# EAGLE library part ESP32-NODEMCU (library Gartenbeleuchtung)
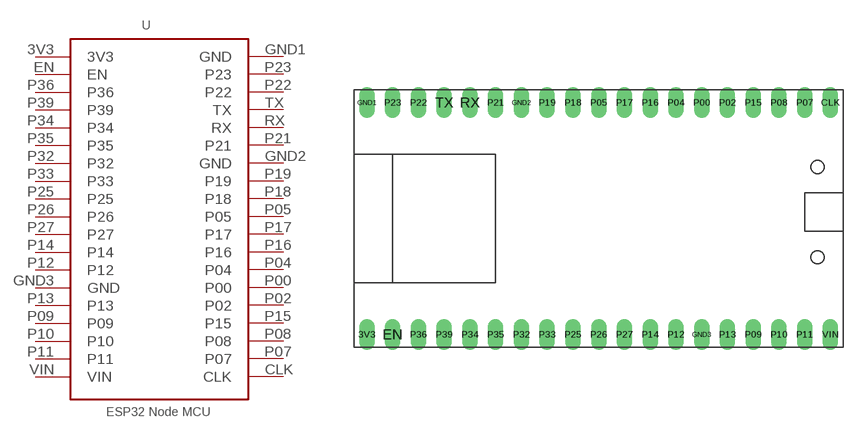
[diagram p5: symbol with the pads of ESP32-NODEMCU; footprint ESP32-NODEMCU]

Designator prefix -

## ESP32-NODEMCU  [ESP32-NODEMCU]
3V3  3V3  pwr
CLK  CLK
EN  EN
GND1  GND  pwr
GND2  GND  pwr
GND3  GND  pwr
P00  P00
P02  P02
P04  P04
P05  P05
P07  P07
P08  P08
P09  P09
P10  P10
P11  P11
P12  P12
P13  P13
P14  P14
P15  P15
P16  P16
P17  P17
P18  P18
P19  P19
P21  P21
P22  P22
P23  P23
P25  P25
P26  P26
P27  P27
P32  P32
P33  P33
P34  P34
P35  P35
P36  P36
P39  P39
RX  RX
TX  TX
VIN  VIN  pwr

## Footprint ESP32-NODEMCU (pad centres in mm)
drill 1 pad 1.422 long: 3V3 -22.86,-12.7; CLK 22.86,10.16; EN -20.32,-12.7; GND1 -22.86,10.16; GND2 -7.62,10.16; GND3 10.16,-12.7; P00 10.16,10.16; P02 12.7,10.16; P04 7.62,10.16; P05 0,10.16; P07 20.32,10.16; P08 17.78,10.16; P09 15.24,-12.7; P10 17.78,-12.7; P11 20.32,-12.7; P12 7.62,-12.7; P13 12.7,-12.7; P14 5.08,-12.7; P15 15.24,10.16; P16 5.08,10.16; P17 2.54,10.16; P18 -2.54,10.16; P19 -5.08,10.16; P21 -10.16,10.16; P22 -17.78,10.16; P23 -20.32,10.16; P25 -2.54,-12.7; P26 0,-12.7; P27 2.54,-12.7; P32 -7.62,-12.7; P33 -5.08,-12.7; P34 -12.7,-12.7; P35 -10.16,-12.7; P36 -17.78,-12.7; P39 -15.24,-12.7; RX -12.7,10.16; TX -15.24,10.16; VIN 22.86,-12.7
